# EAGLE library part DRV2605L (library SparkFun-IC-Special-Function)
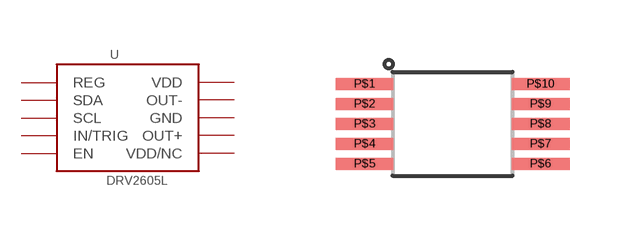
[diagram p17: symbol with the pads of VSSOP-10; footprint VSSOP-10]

Designator prefix -

## DRV2605L (PROD_ID: IC-13504)  [VSSOP-10]
P$1  REG
P$2  SCL
P$3  SDA
P$4  IN/TRIG
P$5  EN
P$6  VDD/NC
P$7  OUT+
P$8  GND
P$9  OUT-
P$10  VDD

## Footprint VSSOP-10 (pad centres in mm)
smd 1.45 x 0.3: P$1 -1.905,1.06; P$2 -1.905,0.56; P$3 -1.905,0.06; P$4 -1.905,-0.44; P$5 -1.905,-0.94; P$6 2.495,-0.94; P$7 2.495,-0.44; P$8 2.495,0.06; P$9 2.495,0.56; P$10 2.495,1.06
